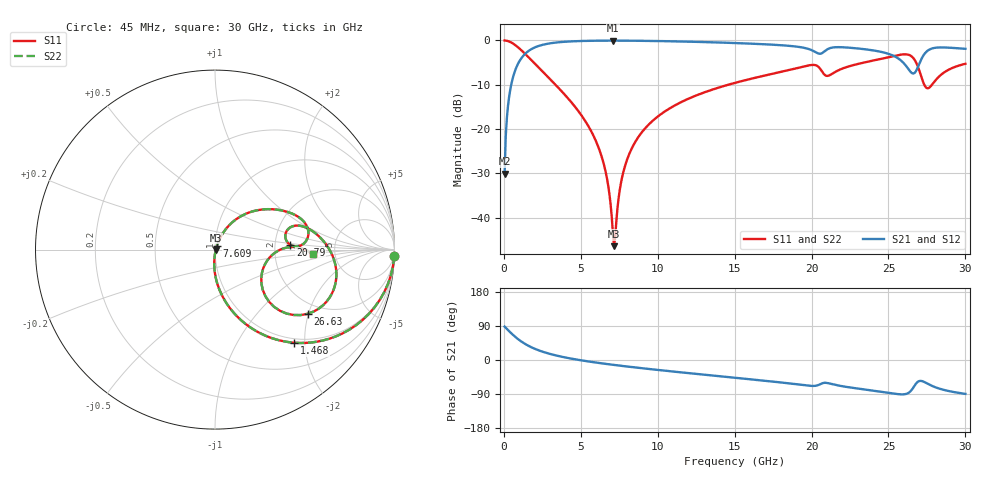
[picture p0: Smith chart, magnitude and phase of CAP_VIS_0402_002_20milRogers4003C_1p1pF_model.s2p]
! S-parameter model data by Modelithics Inc.  support@modelithics.com  813-866-6335  Tampa FL USA
! S-Parameter data specifications:
! Substrate: 20-mil Rogers 4003C, substrate thickness, H=0.508mm, Dielectric constant, Er=3.75
! PCB Mounting Pad Footprint: Pad width, PadW=0.50mm , Pad length, PadL=0.50mm , Pad gap, PadG (edge-to-edge)=0.40mm , Reference planes=1.4mm apart
! Created Wed Nov 18 12:37:07 2015
# hz S ma R 50
! 2 Port Network Data from SP1.SP block
! freq  magS11  angS11  magS21  angS21  magS12  angS12  magS22  angS22
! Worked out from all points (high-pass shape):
!   401 points, 45 MHz to 30 GHz, reference 50 ohm
!   highest |S21| = -0.04 dB at 7.084 GHz (marker M1); lowest = -30.0 dB at 45 MHz (marker M2)
!   |S21| within 3 dB of the highest: 1.372 GHz to 25.02 GHz (23.65 GHz wide, 179 % of centre); 27.34 GHz to end of sweep
!   lowest |S11| = -46.4 dB at 7.159 GHz (marker M3), VSWR 1.01, Z = 50.5 - j0.164 ohm
!   |S11| at or under -10 dB: 3.354 GHz to 14.58 GHz (11.22 GHz wide, 125 % of centre); 27.33 GHz to 27.83 GHz (497.5 MHz wide, 1.8 % of centre)
!   |S22| runs from -46.4 to 0.0 dB; largest |S21 - S12| = 0
!   S11 on the Smith chart (normalised r, x): 45 MHz: 1, -61; 1.468 GHz: 0.92, -1.79; 7.609 GHz: 1.02, +0.04; 20.79 GHz: 2.44, +0.16; 26.63 GHz: 1.67, -1.97; 30 GHz: 3.38, -0.26
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4.5e7  0.9995 -1.9  0.03147 88.1  0.03147 88.1  0.9995 -1.9
2.696625e8  0.9826 -11.2  0.1856 78.8  0.1856 78.8  0.9826 -11.2
4.94325e8  0.9445 -20.1  0.3282 69.9  0.3282 69.9  0.9445 -20.1
1.467862e9  0.6817 -49.6  0.73 40.3  0.73 40.3  0.6817 -49.6
2.890725e9  0.3827 -72.4  0.921 17.2  0.921 17.2  0.3827 -72.4
5.062462e9  0.1411 -89.5  0.9859 -1.1  0.9859 -1.1  0.1411 -89.5
6.410438e9  0.04541 -93.5  0.9943 -9.1  0.9943 -9.1  0.04541 -93.5
6.784875e9  0.02276 -89.4  0.9949 -11.1  0.9949 -11.1  0.02276 -89.4
7.084425e9  0.006749 -58.3  0.9951 -12.7  0.9951 -12.7  0.006749 -58.3
7.159312e9  0.004781 -19.9  0.995 -13.0  0.995 -13.0  0.004781 -19.9
7.608638e9  0.02464 63.2  0.9946 -15.3  0.9946 -15.3  0.02464 63.2
8.4324e9  0.06653 66.3  0.9923 -19.2  0.9923 -19.2  0.06653 66.3
1.007992e10  0.142 61.1  0.9838 -26.6  0.9838 -26.6  0.142 61.1
1.50225e10  0.3322 41.8  0.9349 -46.9  0.9349 -46.9  0.3322 41.8
2.003996e10  0.5297 13.0  0.7721 -68.4  0.7721 -68.4  0.5297 13.0
2.078884e10  0.4204 3.6  0.741 -60.5  0.741 -60.5  0.4204 3.6
2.22117e10  0.4963 15.4  0.8339 -70.7  0.8339 -70.7  0.4963 15.4
2.505742e10  0.651 -2.2  0.7007 -86.9  0.7007 -86.9  0.651 -2.2
2.603096e10  0.6977 -16.8  0.5449 -90.4  0.5449 -90.4  0.6977 -16.8
2.663006e10  0.6274 -34.8  0.4239 -71.8  0.4239 -71.8  0.6274 -34.8
2.752871e10  0.2883 -21.6  0.7624 -62.2  0.7624 -62.2  0.2883 -21.6
3e10  0.5454 -2.8  0.8048 -89.4  0.8048 -89.4  0.5454 -2.8
